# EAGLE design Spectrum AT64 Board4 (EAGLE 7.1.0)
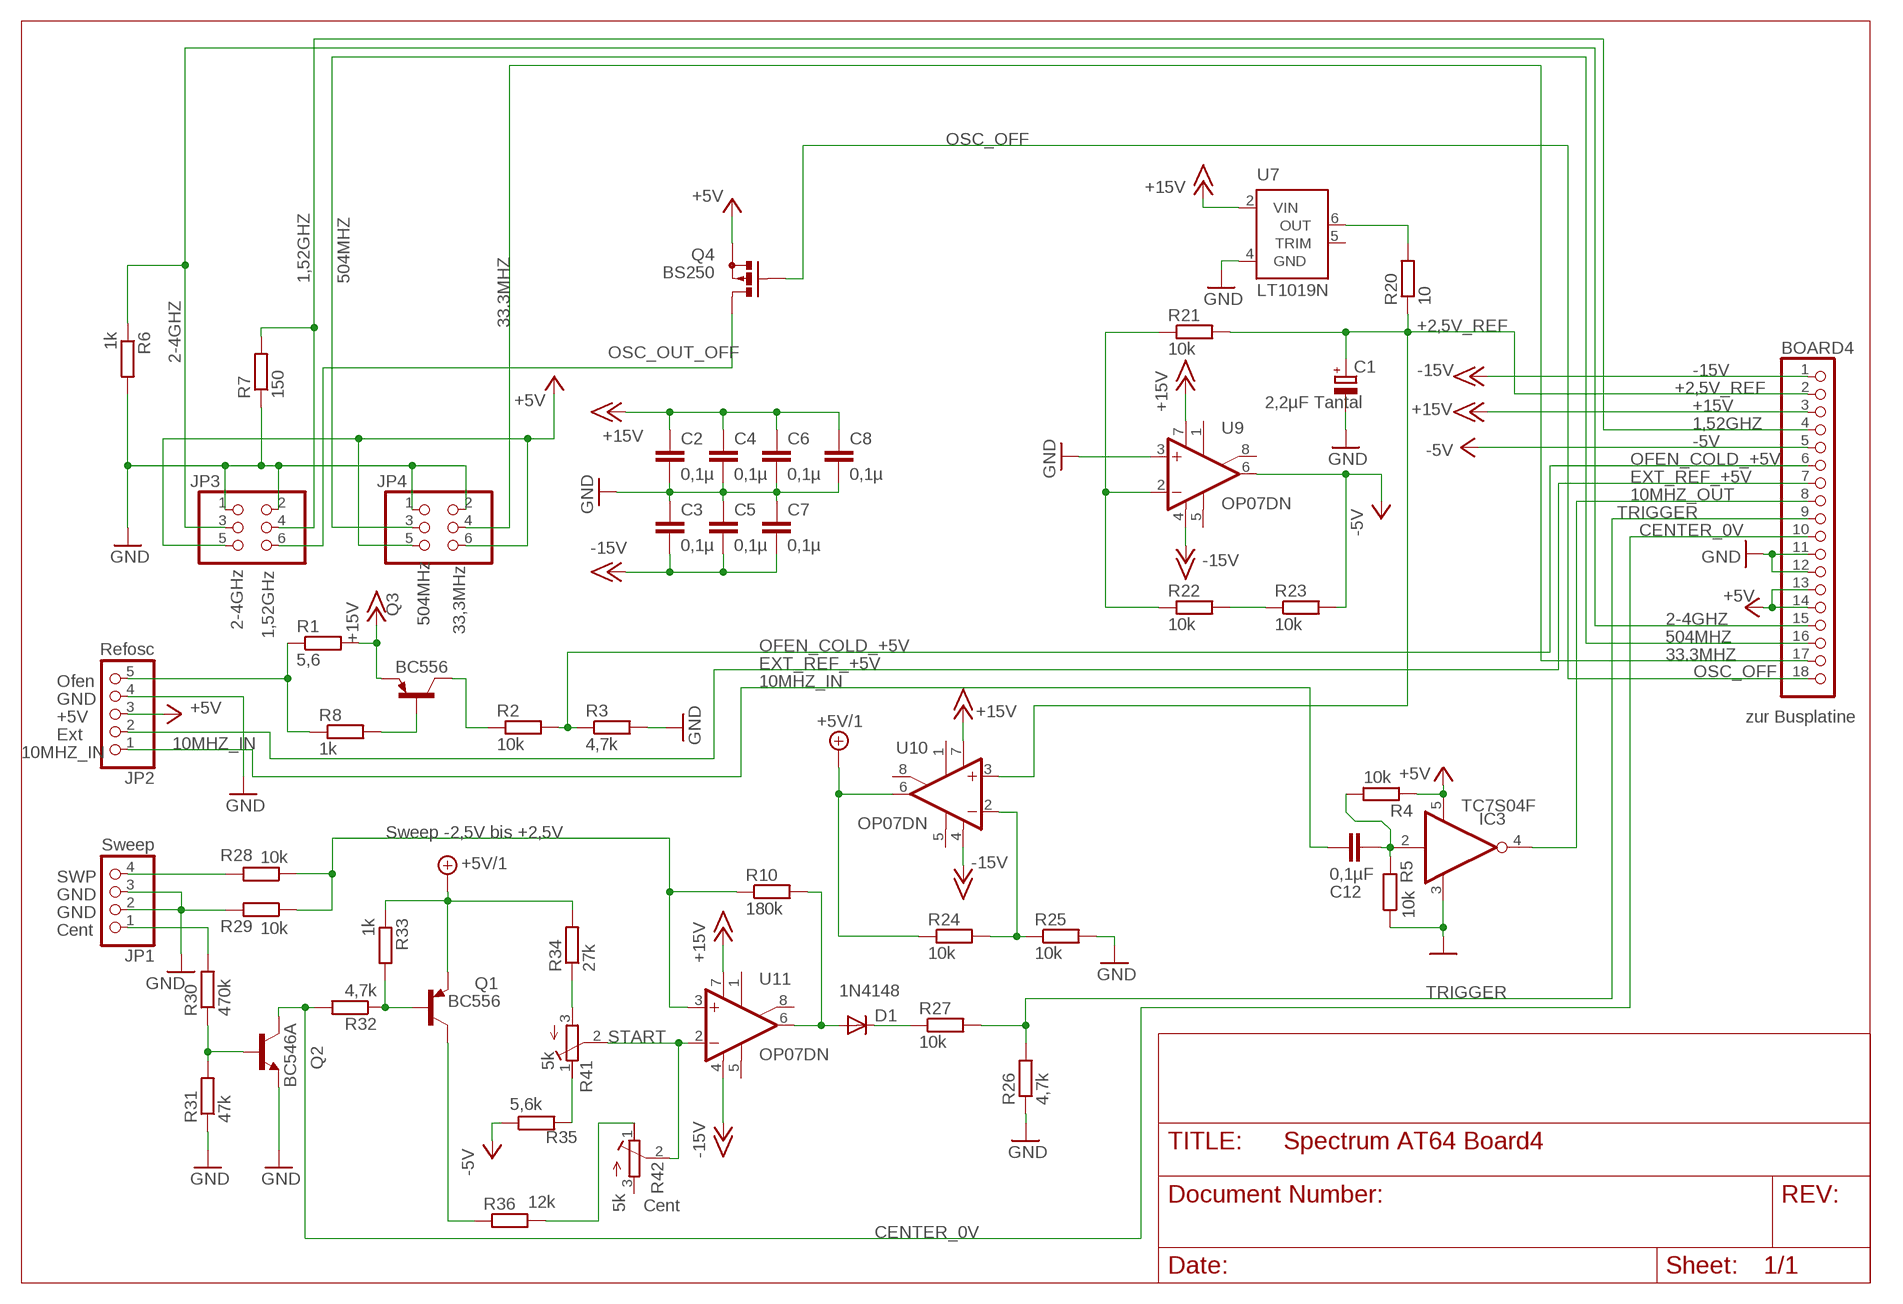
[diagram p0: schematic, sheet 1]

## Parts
BOARD4  zur Busplatine  PINHD-1X18_2.54-90°  [1X18/90]
C1  2,2µF Tantal  CPOL-EUE2.5-5  [E2,5-5]
C2  0,1µ  C5/2.5  [C5B2.5]
C3  0,1µ  C5/2.5  [C5B2.5]
C4  0,1µ  C5/2.5  [C5B2.5]
C5  0,1µ  C5/2.5  [C5B2.5]
C6  0,1µ  C5/2.5  [C5B2.5]
C7  0,1µ  C5/2.5  [C5B2.5]
C8  0,1µ  C5/2.5  [C5B2.5]
C12  0,1µF  C-EUC0805  [C0805]
D1  1N4148  1N4148DO35-7  [DO35-7]
IC3  TC7S04F  [SSOP5]
JP1  Sweep  PINHD-1X04_2.54-90°-S  [1X04/90-S]
JP2  Refosc  PINHD-1X05_2.54-90°  [1X05/90]
JP3  PINHD-2X03_2.54-90°  [2X03/90]
JP4  PINHD-2X03_2.54-90°  [2X03/90]
Q1  BC556  [TO92-EBC]
Q2  BC546A  [TO92-EBC]
Q3  BC556  [TO92-EBC]
Q4  BS250  [SOT54E]
R1  5,6  WIDERSTAND_10  [207.10]
R2  10k  WIDERSTAND_10  [207.10]
R3  4,7k  WIDERSTAND_10  [207.10]
R4  10k  R-EU_R0805  [R0805]
R5  10k  R-EU_R0805  [R0805]
R6  1k  WIDERSTAND_10  [207.10]
R7  150  WIDERSTAND_10  [207.10]
R8  1k  WIDERSTAND_10  [207.10]
R10  180k  R-EU_R0805  [R0805]
R20  10  WIDERSTAND_10  [207.10]
R21  10k  WIDERSTAND_10  [207.10]
R22  10k  WIDERSTAND_10  [207.10]
R23  10k  WIDERSTAND_10  [207.10]
R24  10k  WIDERSTAND_10  [207.10]
R25  10k  WIDERSTAND_10  [207.10]
R26  4,7k  WIDERSTAND_10  [207.10]
R27  10k  WIDERSTAND_10  [207.10]
R28  10k  WIDERSTAND_10  [207.10]
R29  10k  WIDERSTAND_10  [207.10]
R30  470k  WIDERSTAND_10  [207.10]
R31  47k  WIDERSTAND_10  [207.10]
R32  4,7k  WIDERSTAND_10  [207.10]
R33  1k  WIDERSTAND_10  [207.10]
R34  27k  WIDERSTAND_10  [207.10]
R35  5,6k  WIDERSTAND_10  [207.10]
R36  12k  WIDERSTAND_10  [207.10]
R41  5k  R-TRIMM43P  [RTRIM43P]
R42  5k  R-TRIMM43P  [RTRIM43P]
U7  LT1019N  [DIL08]
U9  OP07DN  [DIL08]
U10  OP07DN  [DIL08]
U11  OP07DN  [DIL08]

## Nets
1,52GHZ: BOARD4.4 JP3.4 R7.2
2-4GHZ: BOARD4.15 JP3.3 R6.1
10MHZ_IN: C12.2 JP2.1
10MHZ_OUT: BOARD4.8 IC3.4(O)
33.3MHZ: BOARD4.17 JP4.4
504MHZ: BOARD4.16 JP4.3
+2,5V_REF: BOARD4.2 C1.+ R20.1 R21.2 U10.3(+IN)
+5V: BOARD4.13 BOARD4.14 IC3.5(VCC) JP2.3 JP3.5 JP4.5 JP4.6 Q4.S R4.2
+5V/1: Q1.E R24.1 R33.1 R34.2 U10.6(OUT)
+15V: BOARD4.3 C2.1 C4.1 C6.1 C8.1 Q3.E R1.2 U7.2(VIN) U9.7(V+) U10.7(V+) U11.7(V+)
-5V: BOARD4.5 R23.2 R35.1 U9.6(OUT)
-15V: BOARD4.1 C3.2 C5.2 C7.2 U9.4(V-) U10.4(V-) U11.4(V-)
CENTER_0V: BOARD4.10 Q2.C R32.2
EXT_REF_+5V: BOARD4.7 JP2.2
GND: BOARD4.11 BOARD4.12 C1.- C2.2 C3.1 C4.2 C5.1 C6.2 C7.1 C8.2 IC3.3(GND) JP1.2 JP1.3 JP2.4 JP3.1 JP3.2 JP4.1 JP4.2 Q2.E R3.2 R5.1 R6.2 R7.1 R25.2 R26.1 R29.2 R31.1 U7.4(GND) U9.3(+IN)
N$1: Q3.B R8.2
N$5: JP1.4 R28.2
N$7: JP1.1 R30.2
N$8: Q2.B R30.1 R31.2
N$9: C12.1 IC3.2(I) R4.1 R5.2
N$10: Q1.B R32.1 R33.2
N$11: R10.1 R28.1 R29.1 U11.3(+IN)
N$12: Q1.C R36.1
N$13: R36.2 R42.1(A)
N$14: R34.1 R41.3(E)
N$15: R35.2 R41.1(A)
N$17: R24.2 R25.1 U10.2(-IN)
N$18: D1.A R10.2 U11.6(OUT)
N$19: D1.C R27.1
N$22: JP2.5 R1.1 R8.1
N$24: R22.2 R23.1
N$25: R21.1 R22.1 U9.2(-IN)
N$27: R20.2 U7.6(OUT)
N$31: Q3.C R2.1
OFEN_COLD_+5V: BOARD4.6 R2.2 R3.1
OSC_OFF: BOARD4.18 Q4.G
OSC_OUT_OFF: JP3.6 Q4.D
START: R41.2(S) R42.2(S) U11.2(-IN)
TRIGGER: BOARD4.9 R26.2 R27.2
Unconnected: R42.3(E) U7.5(TRIM) U9.1(ON1) U9.5(OPT) U9.8(ON2) U10.1(ON1) U10.5(OPT) U10.8(ON2) U11.1(ON1) U11.5(OPT) U11.8(ON2)

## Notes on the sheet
- 2-4GHz | 504MHz
- 1,52GHz | 33,3MHz
- Ofen
- GND
- +5V
- Ext
- Sweep -2,5V bis +2,5V
- SWP
- GND
- GND
- Cent
- Cent

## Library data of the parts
BOARD4 = pinhead-2:PINHD-1X18: PIN HEADER
C1 = rcl:CPOL-EU: POLARIZED CAPACITOR, European symbol
C2-C8 = capacitor-wima:C: CAPACITOR
C12 = rcl:C-EU: CAPACITOR, European symbol
D1 = diode:1N4148: DIODE
IC3 = 1Eigene:TC7S04F
JP1 = pinhead-2:PINHD-1X04: PIN HEADER
JP2 = pinhead-2:PINHD-1X05: PIN HEADER
JP3 JP4 = pinhead-2:PINHD-2X03: PIN HEADER
Q1 Q3 = transistor-pnp:BC556*: PNP Transistror
Q2 = transistor-npn:BC546*: NPN Transistor
Q4 = transistor-small-signal:BS250: P-CHANNEL MOS FET
R1-R3 R6-R8 R20-R36 = 1Eigene:WIDERSTAND_10
R4 R5 R10 = rcl:R-EU_: RESISTOR, European symbol
R41 R42 = rcl:R-TRIMM: Trimm resistor
U7 = linear-technology:LT1019?*: Precision Voltage Reference Source: http://www.linear.com/pc/downloadDocument.do?navId=H0,C1,C1154,C1002,C1243,P1130,D3834
U9-U11 = linear:OP07*: OP AMP

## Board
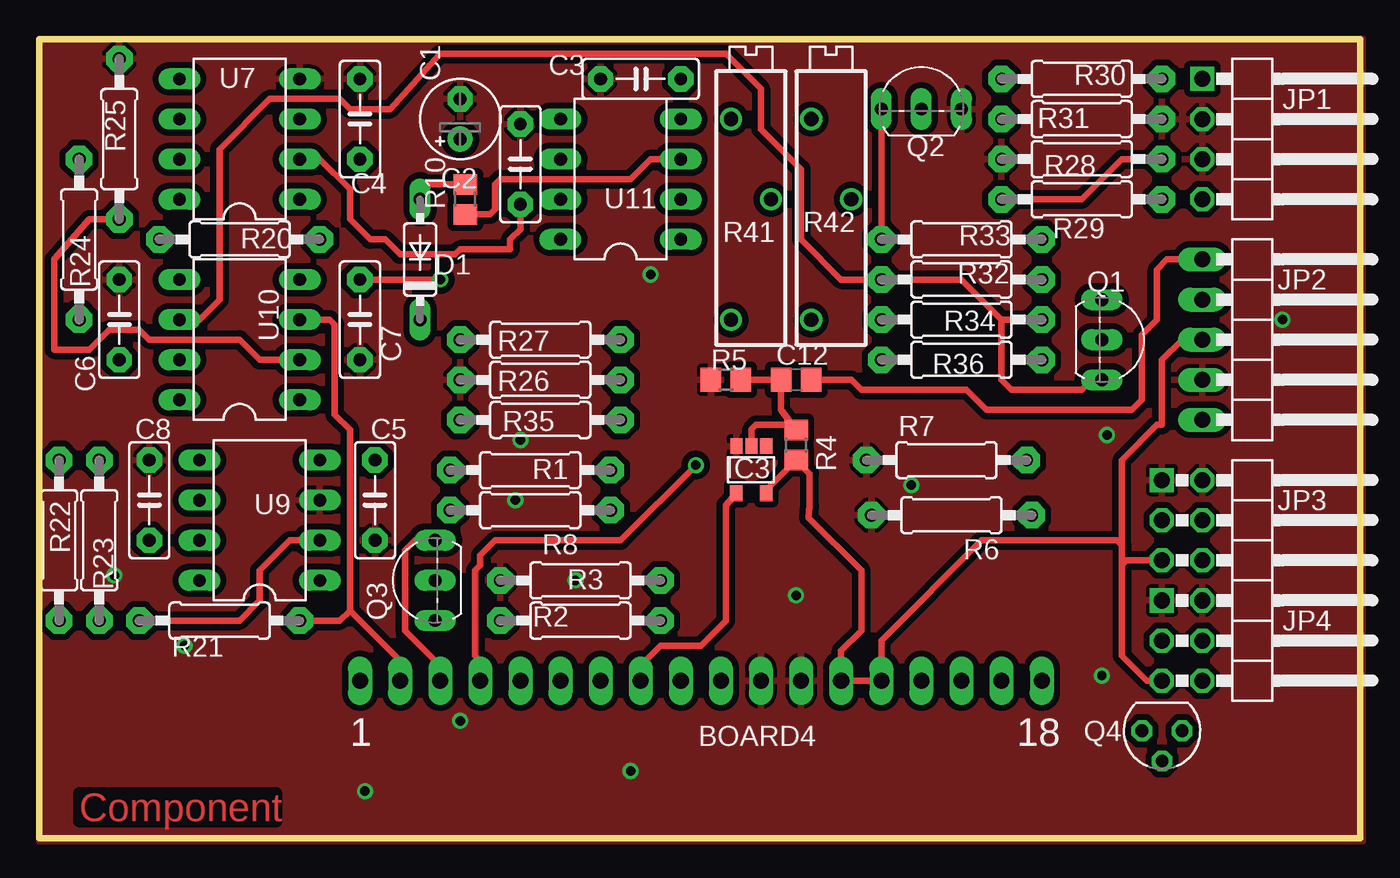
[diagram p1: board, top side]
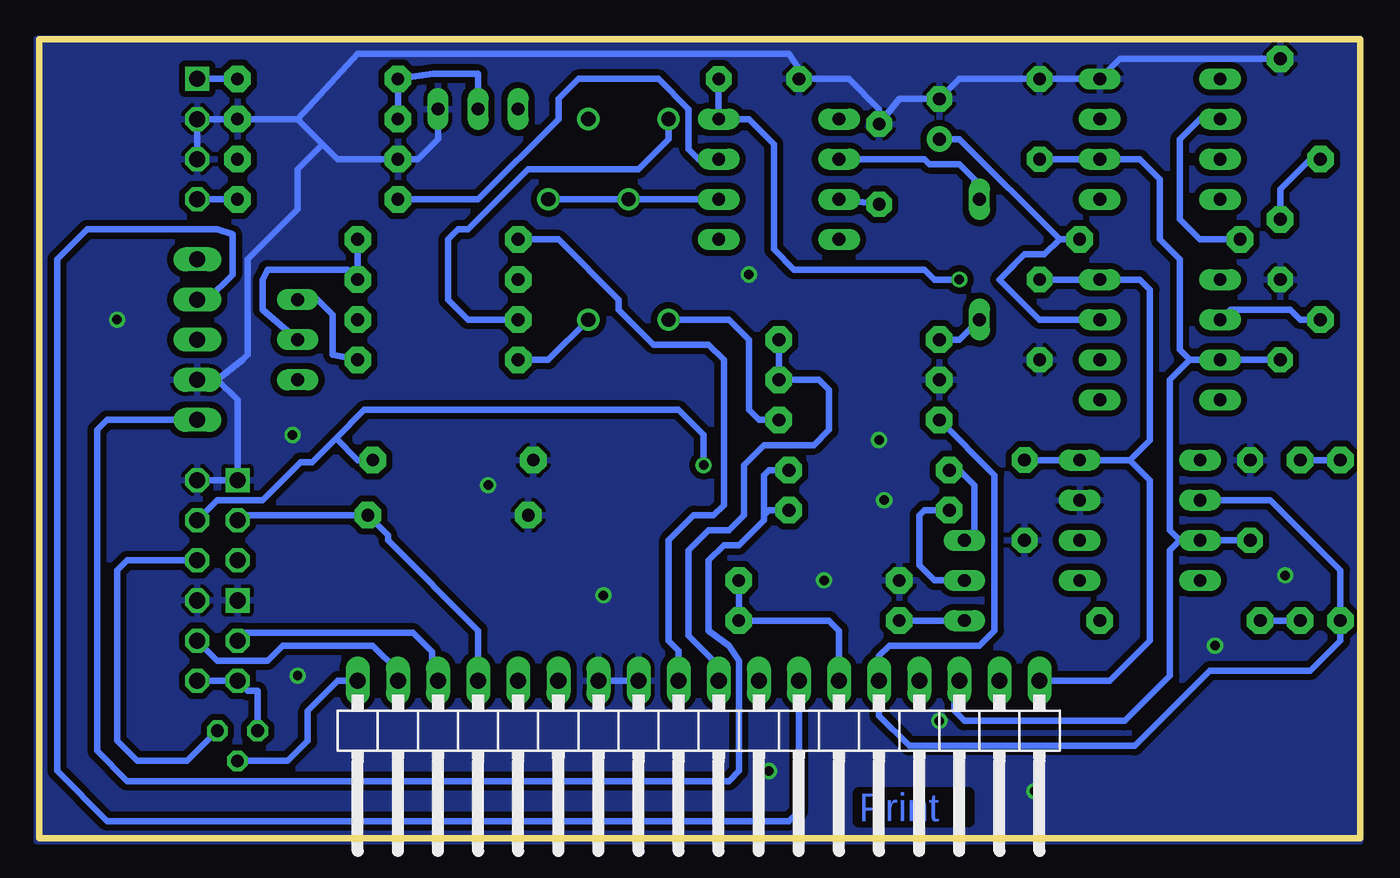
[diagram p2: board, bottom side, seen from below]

Size 83.63 x 50.58 mm. Coordinates in mm from the lower left corner, seen from the top.
Outline: 0,0 83.63,0 83.63,50.58 0,50.58 0,0
Copper layers (1*16): Top 0.035mm / dielectric 1.5mm / Bottom 0.035mm
Design rules "default *": minimum track width 0.4mm, minimum drill 0.6mm, track to track 0.4mm, track to pad 0.3mm, pad to pad 0.4mm, via to via 0.4mm, smd to smd 0.4mm, copper to edge 0mil, drill to drill 0.0152mm, minimum pad ring 10mil, minimum via ring 8mil, stop-mask expansion 4mil, vias tented up to drill 0mil, thermal gap 10mil

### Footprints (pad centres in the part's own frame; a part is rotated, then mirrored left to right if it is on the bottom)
1X18/90 = drill 1.016 long: 1 -21.59,-3.81; 2 -19.05,-3.81; 3 -16.51,-3.81; 4 -13.97,-3.81; 5 -11.43,-3.81; 6 -8.89,-3.81; 7 -6.35,-3.81; 8 -3.81,-3.81; 9 -1.27,-3.81; 10 1.27,-3.81; 11 3.81,-3.81; 12 6.35,-3.81; 13 8.89,-3.81; 14 11.43,-3.81; 15 13.97,-3.81; 16 16.51,-3.81; 17 19.05,-3.81; 18 21.59,-3.81
E2,5-5 = drill 0.813 pad 1.6: + -1.27,0 | drill 0.813 pad 1.6 octagon: - 1.27,0
C5B2.5 = drill 0.813 pad 1.6 octagon: 1 -2.54,0; 2 2.54,0
C0805 = smd 1.3 x 1.5: 1 -0.95,0; 2 0.95,0
DO35-7 = drill 0.813 long: A 3.81,0; C -3.81,0
SSOP5 = smd 0.787 x 0.991: 1 0.965,1.518; 2 0.036,1.518; 3 -0.914,1.518; 4 -0.925,-1.469; 5 0.975,-1.469
1X04/90-S = drill 1.016 square: 1 -3.81,-3.81 | drill 1.016 octagon: 2 -1.27,-3.81; 3 1.27,-3.81; 4 3.81,-3.81
1X05/90 = drill 1.016 long: 1 -5.08,-3.81; 2 -2.54,-3.81; 3 0,-3.81; 4 2.54,-3.81; 5 5.08,-3.81
2X03/90 = drill 1.016 square: 1 -2.54,-6.35 | drill 1.016 octagon: 2 -2.54,-3.81; 3 0,-6.35; 4 0,-3.81; 5 2.54,-6.35; 6 2.54,-3.81
TO92-EBC = drill 0.813 long: B 0,-1.27; C -2.54,-1.27; E 2.54,-1.27
SOT54E = drill 0.813 octagon: D -1.27,0; G 0,1.905; S 1.27,0
207.10 = drill 0.813 pad 1.676 octagon: 1 -5.08,0; 2 5.08,0
R0805 = smd 1.3 x 1.5: 1 -0.95,0; 2 0.95,0
RTRIM43P = drill 0.9: 1 -7.62,1.27; 2 0,-1.27; 3 5.08,1.27
DIL08 = drill 0.813 long: 1 -3.81,-3.81; 2 -1.27,-3.81; 3 1.27,-3.81; 4 3.81,-3.81; 5 3.81,3.81; 6 1.27,3.81; 7 -1.27,3.81; 8 -3.81,3.81

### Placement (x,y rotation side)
BOARD4  41.88,6.17 180 bottom
C1  26.64,45.54 90 top
C2  30.45,42.68 90 top
C3  38.07,48.08 0 top
C4  20.29,45.54 90 top
C5  21.25,21.41 90 top
C6  5.05,32.84 90 top
C7  20.29,32.84 90 top
C8  6.96,21.41 90 top
C12  47.92,29.03 0 top
D1  24.1,36.65 90 top
IC3  45.06,23.32 0 top
JP1  77.44,44.27 270 top
JP2  77.44,31.57 270 top
JP3  77.44,20.14 270 top
JP4  77.44,12.52 270 top
Q1  68.55,31.57 270 top
Q2  55.85,47.45 0 top
Q3  23.79,16.33 90 top
Q4  71.09,6.81 180 top
R1  31.09,23.32 180 top
R2  34.26,13.79 0 top
R3  34.26,16.33 180 top
R4  47.92,24.9 270 top
R5  43.47,29.03 0 top
R6  57.76,20.46 180 top
R7  57.44,23.95 0 top
R8  31.09,20.78 180 top
R10  26.96,40.46 90 top
R20  12.67,37.92 180 top
R21  11.4,13.79 0 top
R22  3.78,18.87 90 top
R23  1.24,18.87 270 top
R24  2.51,37.92 90 top
R25  5.05,44.27 90 top
R26  31.72,29.03 0 top
R27  31.72,31.57 0 top
R28  66.01,40.46 0 top
R29  66.01,43 180 top
R30  66.01,48.08 0 top
R31  66.01,45.54 180 top
R32  58.39,37.92 180 top
R33  58.39,35.38 0 top
R34  58.39,32.84 0 top
R35  31.72,26.49 0 top
R36  58.39,30.3 180 top
R41  45.06,40.46 90 top
R42  50.14,40.46 90 top
U7  12.67,44.27 90 top
U9  13.94,20.14 90 top
U10  12.67,31.57 90 top
U11  36.8,41.73 90 top

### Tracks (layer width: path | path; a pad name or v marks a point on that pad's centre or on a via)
1,52GHZ  (via drill 0.6 pad 1.02)
  Top 0.406: v41.57,23.63 36.8,18.87 28.87,18.87 27.91,17.92 27.91,17.28 27.6,16.97 27.6,11.57 27.91,11.25 BOARD4.4
  Bottom 0.406: v41.57,23.63 41.57,25.54 43.15,27.13 63.07,27.13 64.86,25.34 | 64.86,25.34 66.37,23.82 67.1,23.82 69.51,21.41 72.36,21.41 JP3.4 | R7.2 63.47,23.95 64.86,25.34
2-4GHZ
  Bottom 0.406: BOARD4.15 55.85,13.16 61.57,18.87 61.57,19.19 R6.1 70.78,20.46 JP3.3
10MHZ_IN
  Top 0.406: C12.2 51.41,29.03 52.04,28.4 58.71,28.4 59.98,27.13 69.19,27.13 69.82,27.76 69.82,31.89 70.78,32.84 70.78,36.02 71.41,36.65 JP2.1
10MHZ_OUT
  Top 0.406: BOARD4.8 38.07,10.94 39.34,12.21 41.88,12.21 43.47,13.79 43.47,21.1 44.11,21.82 IC3.4
33.3MHZ
  Bottom 0.406: BOARD4.17 60.93,10.62 62.52,12.21 68.24,12.21 69.19,11.25 72.36,11.25 JP4.4
504MHZ
  Bottom 0.4: BOARD4.16 58.77,10.22 58.77,11.82 59.97,13.02 70.77,13.02 71.17,12.62 JP4.3
+2,5V_REF
  Top 0.4: 18.71,26.81 18.71,32.53 18.39,32.84 U10.3
  Top 0.406: 18.71,26.81 19.66,25.86 19.66,14.43 | 19.66,14.43 19.02,13.79 R21.2 | BOARD4.2 22.83,11.25 19.66,14.43
  Bottom 0.4: U10.3 20.29,32.84 22.83,35.38 21.56,36.65
  Bottom 0.406: C1.+ 25.37,44.27 19.02,37.92 | 19.02,37.92 R20.1 | 19.02,37.92 19.98,36.97 21.25,36.97 21.56,36.65 22.2,36.02
+5V
  Top 0.4: 48.77,21.02 48.7,20.31 48.69,20.31
  Top 0.406: JP2.3 72.36,31.57 71.09,30.3 71.09,26.17 70.78,26.17 68.55,23.95 68.55,18.56 | 48.7,20.31 52.04,16.97 52.04,13.16 50.77,11.89 BOARD4.13 BOARD4.14 53.31,12.52 59.66,18.87 68.24,18.87 68.55,18.56 | IC3.5 46.03,22.07 R4.2 48.77,23.1 48.77,21.02 | 68.55,17.28 68.55,11.57 70.14,9.98 JP4.5 | 68.55,18.56 68.55,17.28 | JP3.5 68.87,17.6 68.55,17.28
  Bottom 0.406: Q4.S 69.82,9.35 70.46,9.35 JP4.5 JP4.6
+5V/1
  Top 0.406: U10.6 10.13,32.84 11.4,34.11 11.4,43.64 14.58,46.81 19.02,46.81 19.66,46.18 22.2,46.18 25.37,49.67 43.47,49.67 45.69,47.45 45.69,44.91 48.23,42.37 48.23,37.92 50.77,35.38 R33.1 58.39,35.38 60.93,32.84 | 60.93,32.84 R34.2 | Q1.E 66.65,29.03 66.01,28.4 61.57,28.4 60.93,29.03 60.93,32.84
  Bottom 0.406: R24.1 3.78,32.84 4.42,33.48 8.23,33.48 U10.6
+15V
  Top 0.406: U7.2 17.75,43 19.66,41.1 19.66,39.19 20.93,37.92 21.88,37.92 22.83,36.97 26.33,36.97 26.64,37.29 29.82,37.29 29.82,37.92 30.45,38.56 C2.1 | BOARD4.3 25.37,10.94 23.15,13.16 23.15,18.24 23.79,18.87 Q3.E
  Bottom 0.406: 11.4,18.87 12.04,18.24 12.04,10.3 14.9,7.44 25.06,7.44 25.69,8.08 25.69,9.66 BOARD4.3 | 11.4,18.87 U9.7 C8.1 | 11.4,18.87 12.04,19.51 12.04,29.03 10.77,30.3 | 10.77,30.3 U10.7 C6.1 | 10.77,30.3 11.4,30.94 11.4,36.65 12.67,37.92 12.67,41.73 13.94,43 U7.2 C4.1 | U11.7 C2.1 | R1.2 25.37,23.32 24.42,22.37 24.42,19.51 Q3.E
-5V
  Bottom 0.406: U9.6 5.69,21.41 1.24,16.97 R23.2 1.24,12.52 3.15,10.62 9.5,10.62 14.26,5.85 28.55,5.85 30.45,7.76 BOARD4.5 30.45,11.57 29.82,12.21 24.1,12.21 23.15,13.16 23.15,23 R35.1
-15V  (via drill 0.6)
  Top 0.406: C7.2 v25.37,35.38
  Bottom 0.406: C3.2 U11.4 38.71,45.54 37.12,43.96 37.12,37.29 35.85,36.02 27.6,36.02 26.96,35.38 v25.37,35.38 | 14.58,23.95 13.31,22.68 13.31,12.52 15.85,9.98 BOARD4.1 | 14.58,23.95 U9.4 C5.2 | C7.2 U10.4 13.94,35.38 13.31,34.75 13.31,25.22 14.58,23.95
CENTER_0V
  Top 0.406: R32.2 Q2.C
  Bottom 0.406: R32.2 50.77,37.92 46.96,34.11 46.96,33.48 44.74,31.26 41.25,31.26 40.3,30.3 40.3,21.1 40.93,20.46 42.2,20.46 43.79,18.87 43.79,12.52 43.15,11.89 BOARD4.10
EXT_REF_+5V
  Bottom 0.406: JP2.2 73,34.11 71.41,35.7 71.41,38.24 72.36,38.56 80.62,38.56 82.52,36.65 82.52,4.27 79.35,1.09 36.17,1.09 35.53,1.73 BOARD4.7
GND  (via drill 0.6 pad 1.02)
  Bottom 0.406: JP1.3 JP1.2 R31.1 67.28,45.54 | 67.28,45.54 65.7,43.96 | 65.7,43.96 64.74,43 R29.2 59.66,43 58.39,44.27 Q2.E | BOARD4.11 BOARD4.12 | R25.2 15.21,49.35 U7.4 C4.2 25.37,48.08 C1.- 29.18,46.81 C2.2 30.45,46.18 32.36,48.08 C3.1 35.53,48.72 36.17,49.67 63.47,49.67 67.28,45.54 | JP3.2 JP3.1 71.09,27.76 72.36,29.03 | 72.36,29.03 JP2.4 | 72.36,29.03 70.78,30.3 70.46,30.62 70.46,36.65 67.28,39.83 67.28,42.37 65.7,43.96
  other vias: 20.61,3 78.71,32.84 33.95,16.33 55.22,22.36 47.92,15.38 67.28,10.3 30.14,21.41 26.64,7.44 9.18,12.2 4.74,16.65 37.44,4.27 67.6,25.54 38.71,35.7 30.45,25.22
  pour Bottom: -0.03,50.62 83.79,50.62 83.79,-0.18 -0.03,-0.18
  pour Top: -0.03,50.62 83.79,50.62 83.79,-0.18 -0.03,-0.18
N$1
  Bottom 0.406: Q3.B 26.96,16.33 27.91,17.28 27.91,20.46 27.6,20.78 R8.2
N$5
  Bottom 0.406: R28.2 JP1.4
N$7
  Bottom 0.406: R30.2 JP1.1
N$8
  Bottom 0.406: R31.2 R30.1 58.71,48.4 55.85,48.4 Q2.B
N$9
  Top 0.406: IC3.2 45.1,25.89 45.38,26.17 47.6,26.17 R4.1 46.96,27.13 C12.1 R5.2
N$10
  Bottom 0.406: R32.1 R33.2 64.11,36.02 69.19,36.02 69.51,35.38 69.51,33.48 Q1.B
N$11
  Top 0.406: R28.1 66.01,40.46 68.55,43 R29.1 | R10.1 28.55,39.51 28.87,39.83 28.87,41.42 29.18,41.73 37.44,41.73 38.71,43 U11.3
  Bottom 0.406: R28.1 55.85,40.46 50.77,45.54 50.77,46.81 49.5,48.08 44.42,48.08 42.52,46.18 42.52,43.64 41.88,43 U11.3
N$12
  Bottom 0.406: R36.1 65.06,30.62 65.06,33.16 66.01,34.11 Q1.C
N$13
  Bottom 0.406: R42.1 51.41,30.3 R36.2
N$14
  Bottom 0.406: R34.1 56.49,32.84 57.76,34.11 57.76,37.92 57.12,38.56 56.49,38.56 52.68,42.37 45.69,42.37 43.79,44.27 R41.3
N$15
  Bottom 0.406: R35.2 38.07,26.49 38.71,27.13 38.71,31.57 39.98,32.84 R41.1
N$17
  Top 0.406: R25.1 3.15,39.19 0.93,36.65 0.93,30.94 3.15,30.94 4.42,32.21 6.32,32.21 6.96,31.57 12.67,31.57 13.94,30.3 U10.2
  Bottom 0.406: R24.2 3.15,43 5.05,41.1 R25.1
N$18
  Top 0.406: R10.2 24.74,41.41 24.42,41.1 24.42,40.78 D1.A
  Bottom 0.406: U11.6 27.6,43 27.28,42.68 25.37,42.68 24.42,41.73 24.42,40.78 D1.A
N$19
  Bottom 0.406: R27.1 25.37,31.57 D1.C
N$22
  Bottom 0.406: JP2.5 79.35,26.49 79.98,25.86 79.98,5.54 78.08,3.63 39.98,3.63 39.34,4.27 39.34,11.25 39.98,12.21 41.25,13.16 41.25,17.6 40.3,18.56 39.34,18.56 37.76,20.14 37.76,20.46 | 37.76,20.46 37.76,23 37.44,23.32 R1.1 | R8.1 37.44,20.78 37.76,20.46
N$24
  Bottom 0.406: R23.1 R22.2
N$25
  Top 0.406: U9.2 15.85,18.87 13.94,16.97 13.94,15.06 12.67,13.79 R21.1
  Bottom 0.406: R22.1 R21.1
N$27
  Bottom 0.406: U7.6 10.13,45.54 11.4,44.27 11.4,39.19 10.13,37.92 R20.2
N$31
  Bottom 0.406: Q3.C R2.1
OFEN_COLD_+5V
  Bottom 0.406: BOARD4.6 32.99,13.16 33.63,13.79 R2.2 R3.1
OSC_OFF
  Bottom 0.406: Q4.G 67.92,4.9 66.65,6.17 66.65,8.08 64.74,9.98 BOARD4.18
OSC_OUT_OFF
  Bottom 0.406: Q4.D 74.27,4.9 77.44,4.9 78.71,6.17 78.71,16.97 78.08,17.6 JP3.6
START
  Bottom 0.406: R42.2 R41.2 U11.2
TRIGGER
  Bottom 0.406: BOARD4.9 40.93,9.98 40.93,11.25 42.52,12.84 42.52,18.24 41.25,19.51 39.98,19.51 39.03,20.46 39.03,23.63 37.76,24.9 34.58,24.9 33.63,25.86 33.63,28.4 34.26,29.03 R26.2 R27.2

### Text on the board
Top: Component
Bottom: Print
tNames: 1 | 18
